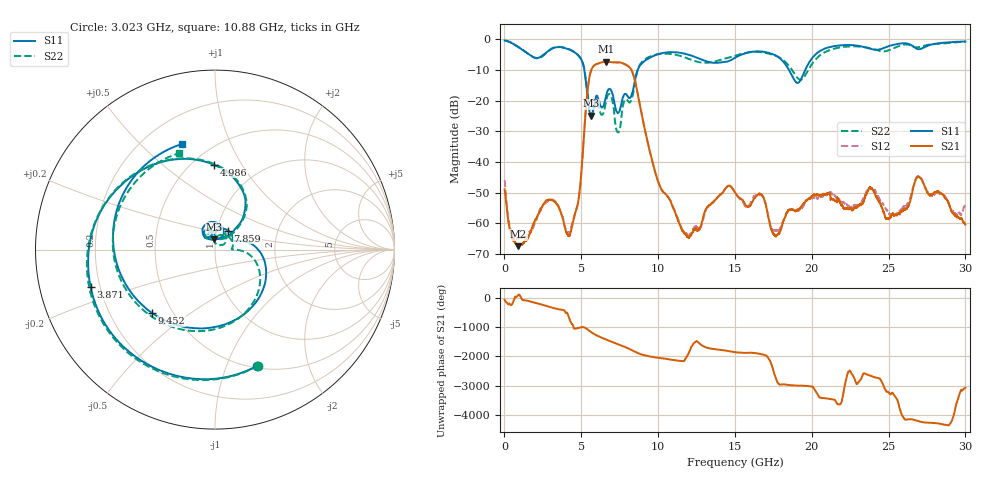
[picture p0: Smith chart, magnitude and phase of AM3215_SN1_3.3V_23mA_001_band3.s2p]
!Agilent Technologies,E8364B,MY43040894,A.07.50.67
!Agilent E8364B: A.07.50.67
!Date: Tuesday, May 25, 2021 15:25:19
!Correction: S11(Full 2 Port(1,2))
!S21(Full 2 Port(1,2))
!S12(Full 2 Port(1,2))
!S22(Full 2 Port(1,2))
!S2P File: Measurements: S11, S21, S12, S22:
# Hz S  dB  R 50
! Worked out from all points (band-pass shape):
!   6401 points, 10 MHz to 30 GHz, reference 50 ohm
!   highest |S21| = -7.30 dB at 6.608 GHz (marker M1); lowest = -67.5 dB at 909.7 MHz (marker M2)
!   |S21| within 3 dB of the highest: 5.63 GHz to 8.291 GHz (2.66 GHz wide, 38.2 % of centre)
!   lowest |S11| = -24.9 dB at 5.633 GHz (marker M3), VSWR 1.12, Z = 49.1 + j5.55 ohm
!   |S11| at or under -10 dB: 5.198 GHz to 8.672 GHz (3.474 GHz wide, 50.1 % of centre); 18.52 GHz to 19.58 GHz (1.059 GHz wide, 5.56 % of centre)
!   |S22| runs from -30.4 to -0.4 dB; largest |S21 - S12| = 0.0087
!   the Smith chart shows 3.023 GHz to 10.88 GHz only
!   S11 on the Smith chart (normalised r, x): 3.023 GHz: 0.52, -1.29; 3.871 GHz: 0.16, -0.14; 4.986 GHz: 0.63, +0.76; 7.859 GHz: 1.13, +0.24; 9.452 GHz: 0.38, -0.36; 10.88 GHz: 0.35, +0.67
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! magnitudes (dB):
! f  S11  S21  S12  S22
! 10 MHz  -0.4  -48.9  -45.9  -0.4
! 909.7 MHz  -2.6  -67.5  -64.9  -2.5
! 3.023 GHz  -3.2  -52.4  -52.3  -3.2
! 3.871 GHz  -2.8  -60.0  -59.3  -2.7
! 4.302 GHz  -3.5  -63.0  -62.5  -3.5
! 4.986 GHz  -6.5  -44.6  -44.9  -6.4
! 5.01 GHz  -6.7  -43.3  -43.5  -6.6
! 5.633 GHz  -24.9  -10.3  -10.3  -24.8
! 6.608 GHz  -18.7  -7.3  -7.3  -20.2
! 7.39 GHz  -24.1  -7.5  -7.6  -30.4
! 7.859 GHz  -17.8  -8.2  -8.2  -19.7
! 9.452 GHz  -6.1  -36.4  -36.5  -5.7
! 10.01 GHz  -4.9  -46.6  -46.5  -4.9
! 10.88 GHz  -4.2  -53.9  -53.6  -4.8
! 12.01 GHz  -5.1  -64.8  -63.7  -6.4
! 15.01 GHz  -6.0  -49.9  -49.9  -5.4
! 16.73 GHz  -4.0  -50.6  -51.0  -4.2
! 17.66 GHz  -5.3  -64.1  -62.3  -5.4
! 20 GHz  -6.3  -51.2  -51.7  -8.2
! 25 GHz  -2.2  -58.7  -56.4  -3.6
! 26.96 GHz  -3.2  -44.8  -44.7  -2.6
! 30 GHz  -0.7  -60.5  -53.7  -0.8
